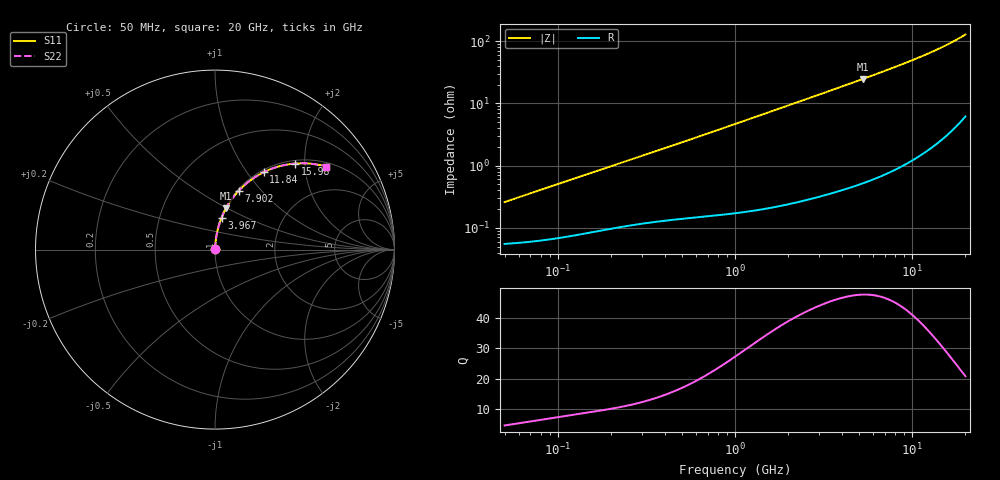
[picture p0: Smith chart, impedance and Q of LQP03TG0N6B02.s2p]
!Murata Part Number: LQP03TG0N6B02
!These Parameters are Measured in Series Mode Connection
!  o--[Z]--o
!Port1  Port2
!  o-------o
!Freq. Start=50[MHz] Stop=20[GHz], 401[Steps]
# Hz S RI R 50
!Freq.(Hz) S11(Real) S11(Imag) S21(Real) S21(Imag) S12(Real) S12(Imag) S22(Real) S22(Imag)
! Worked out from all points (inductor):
!   401 points, 50 MHz to 20 GHz, reference 50 ohm
!   read as one part in series: L = 806 pH near 51.52 MHz
!   highest Q = 47.5 at 5.273 GHz (marker M1), where L = 745 pH
!   S11 on the Smith chart (normalised r, x): 50 MHz: 1.00, +0.01; 3.967 GHz: 1.01, +0.37; 7.902 GHz: 1.02, +0.76; 11.84 GHz: 1.03, +1.20; 15.98 GHz: 1.06, +1.79; 20 GHz: 1.12, +2.56
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5e7  0.000558 0.00254  0.9994 -0.00254  0.9994 -0.00254  0.000558 0.00254
5.152053e7  0.000561 0.00261  0.9994 -0.00261  0.9994 -0.00261  0.000561 0.00261
1.364002e8  0.000837 0.00676  0.9992 -0.00676  0.9992 -0.00676  0.000837 0.00676
3.721004e8  0.00158 0.0176  0.9984 -0.0176  0.9984 -0.0176  0.00158 0.0176
6.380365e8  0.00238 0.0298  0.9976 -0.0298  0.9976 -0.0298  0.00238 0.0298
1e9  0.00386 0.0463  0.9961 -0.0463  0.9961 -0.0463  0.00386 0.0463
1.714689e9  0.00842 0.0787  0.9916 -0.0787  0.9916 -0.0787  0.00842 0.0787
2.728004e9  0.0185 0.1238  0.9815 -0.1238  0.9815 -0.1238  0.0185 0.1238
3.967106e9  0.0365 0.177  0.9635 -0.177  0.9635 -0.177  0.0365 0.177
5.273168e9  0.0618 0.2304  0.9382 -0.2304  0.9382 -0.2304  0.0618 0.2304
6.311513e9  0.0863 0.2704  0.9137 -0.2704  0.9137 -0.2704  0.0863 0.2704
7.442007e9  0.1172 0.311  0.8828 -0.311  0.8828 -0.311  0.1172 0.311
7.901521e9  0.131 0.3265  0.869 -0.3265  0.869 -0.3265  0.131 0.3265
8.774992e9  0.1588 0.3542  0.8412 -0.3542  0.8412 -0.3542  0.1588 0.3542
9.745021e9  0.1922 0.3822  0.8078 -0.3822  0.8078 -0.3822  0.1922 0.3822
1.082228e10  0.2319 0.4095  0.7681 -0.4095  0.7681 -0.4095  0.2319 0.4095
1.183995e10  0.2717 0.4314  0.7283 -0.4314  0.7283 -0.4314  0.2717 0.4314
1.375312e10  0.3506 0.4621  0.6494 -0.4621  0.6494 -0.4621  0.3506 0.4621
1.597544e10  0.4462 0.4796  0.5538 -0.4796  0.5538 -0.4796  0.4462 0.4796
1.774144e10  0.5223 0.4796  0.4777 -0.4796  0.4777 -0.4796  0.5223 0.4796
1.940974e10  0.5923 0.4689  0.4077 -0.4689  0.4077 -0.4689  0.5923 0.4689
2e10  0.6162 0.4628  0.3838 -0.4628  0.3838 -0.4628  0.6162 0.4628
